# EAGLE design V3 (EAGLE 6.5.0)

## Sheet 1 of 3: FET+Driver
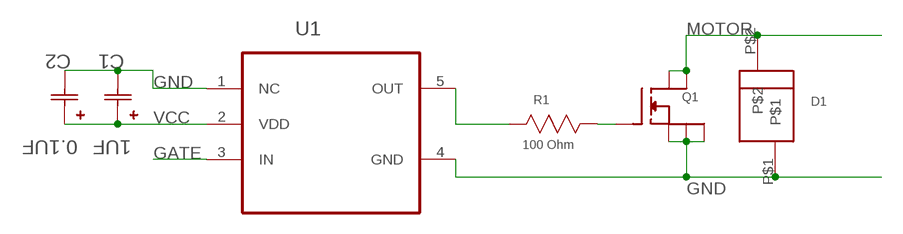
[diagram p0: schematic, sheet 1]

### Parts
C1  1UF  1206YC105KAT2A  [CAPC3216X127N]
C2  0.1UF  0603YC104K4T4A  [CAPC1608X90N]
D1  5.0SMDJ24ASMD  [DO-214AB]
Q1  PSMN039LFPAC  [LFPAC]
R1  100 Ohm  ERA-3AEB101V  [RESC1608X60N]
U1  NCS2001SN1T1G  [SOT95P275X110-5N]

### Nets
GATE: U1.3(IN) ; also sheet 3
GND: C1.2(C2) C2.2(C2) D1.P$1 Q1.1(S1) Q1.2(S2) Q1.3(S3) U1.1(NC) U1.4(GND) ; also sheet 2,3
MOTOR: D1.P$2 Q1.5(D1) Q1.6(D2) ; also sheet 3
N$1: Q1.4(G) R1.1(R1)
N$2: R1.2(R2) U1.5(OUT)
VCC: C1.1(C1) C2.1(C1) U1.2(VDD) ; also sheet 2

## Sheet 2 of 3: Control Power
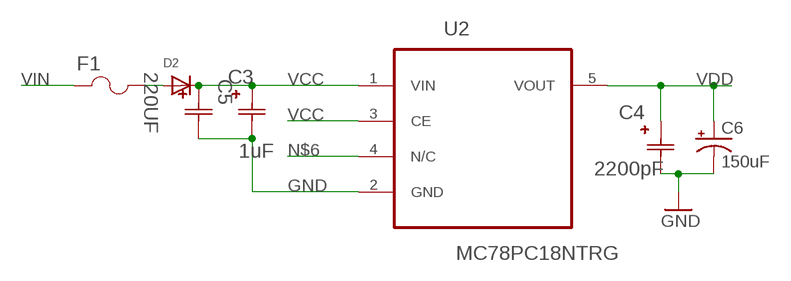
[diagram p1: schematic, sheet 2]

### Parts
C3  1uF  0603YC105KAT2A  [CAPC1608X94N]
C4  2200pF  06033C222JAT4A  [CAPC1608X90N]
C5  220UF  TAJD227K006RNJ  [CAPCP7343X430N]
C6  150uF  47UF-10V-10%(TANT)  [EIA3528]
D2  DIODESOD-123  [SOD-123]
F1  F1206B3R00FWTR  [FUSM3216X140N]
U2  MC78PC18NTRG  [SOT95P275X110-5N]

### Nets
GND: C3.2(C2) C4.2(C2) C5.2(C2) C6.C(-) U2.2(GND) ; also sheet 1,3
N$3: D2.A F1.2
N$6: U2.4(N/C)
VCC: C3.1(C1) C5.1(C1) D2.C U2.1(VIN) U2.3(CE) ; also sheet 1
VDD: C4.1(C1) C6.A(+) U2.5(VOUT) ; also sheet 3
VIN: F1.1

## Sheet 3 of 3: Control + Sensors
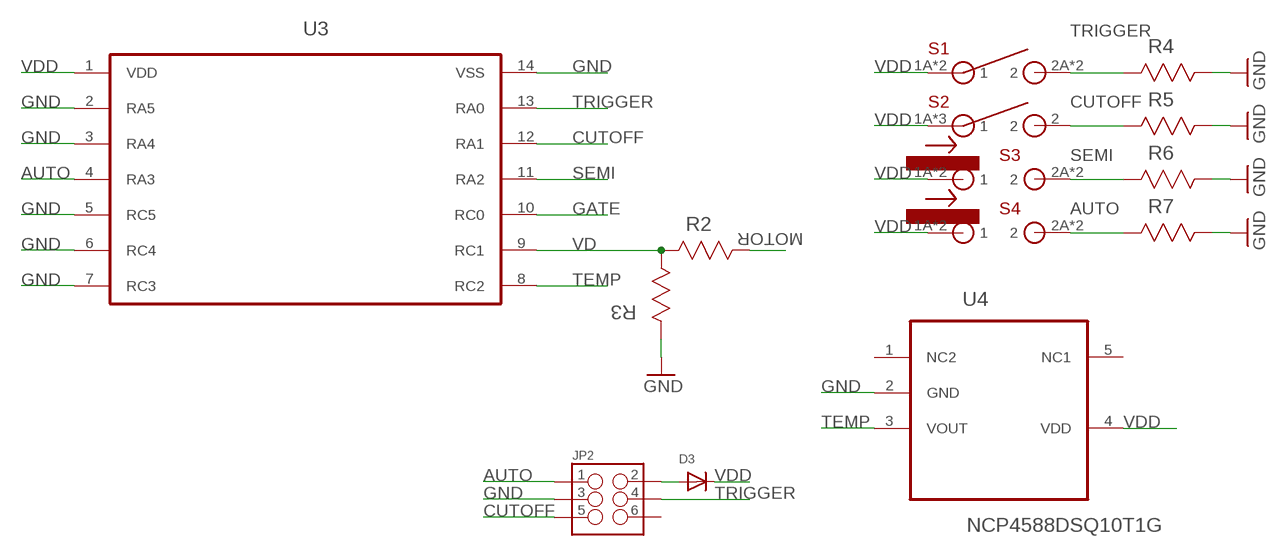
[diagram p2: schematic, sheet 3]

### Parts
D3  DIODESOD-123  [SOD-123]
JP2  M03X2  [2X3_SMD]
R2  15 kOhm  ERA-3AEB153V  [RESC1608X60N]
R3  4.7 kOhm  ERA-3AEB472V  [RESC1608X60N]
R4  4.7 kOhm  ERA-3AEB472V  [RESC1608X60N]
R5  4.7 kOhm  ERA-3AEB472V  [RESC1608X60N]
R6  4.7 kOhm  ERA-3AEB472V  [RESC1608X60N]
R7  4.7 kOhm  ERA-3AEB472V  [RESC1608X60N]
S1  7914S-1-000E  [7914S-1-000E]
S2  ESE-31L15T  [ESE-31L15T]
S3  SPVM110100  [SPVM110100]
S4  SPVM110100  [SPVM110100]
U3  P89LPC912FDH,129  [SOP65P640X110-14N]
U4  NCP4588DSQ10T1G  [SOT65P210X110-5N]

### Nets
AUTO: JP2.1 R7.2(R2) S4.2A S4.2B U3.4(RA3)
CUTOFF: JP2.5 R5.2(R2) S2.2 U3.12(RA1)
GATE: U3.10(RC0) ; also sheet 1
GND: JP2.3 R3.2(R2) R4.1(R1) R5.1(R1) R6.1(R1) R7.1(R1) U3.2(RA5) U3.3(RA4) U3.5(RC5) U3.6(RC4) U3.7(RC3) U3.14(VSS) U4.2(GND) ; also sheet 1,2
MOTOR: R2.1(R1) ; also sheet 1
N$7: D3.A JP2.2
SEMI: R6.2(R2) S3.2A S3.2B U3.11(RA2)
TEMP: U3.8(RC2) U4.3(VOUT)
TRIGGER: JP2.4 R4.2(R2) S1.2A S1.2B U3.13(RA0)
VD: R2.2(R2) R3.1(R1) U3.9(RC1)
VDD: D3.C S1.1A S1.1B S2.1A S2.1B S2.1C S3.1A S3.1B S4.1A S4.1B U3.1(VDD) U4.4(VDD) ; also sheet 2
Unconnected: JP2.6 U4.5(NC1)

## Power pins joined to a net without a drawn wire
NC2: U4.1(NC2)

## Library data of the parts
C1 = AVX_By_element14_Batch_1:1206YC105KAT2A: Capacitor 1206; MPN: 1206YC105KAT2A; OC_FARNELL: 499717; OC_NEWARK: 25C3294; SUPPLIER: AVX; TOLERANCE: ±10%; VOLTAGERATING: 16V
C2 = AVX_By_element14_Batch_1:0603YC104K4T4A: Capacitor, 0603; MPN: 0603YC104K4T4A; OC_FARNELL: 1833863; OC_NEWARK: 85R5663; SUPPLIER: AVX; TOLERANCE: ±10%; VOLTAGERATING: 16V
C3 = AVX_By_element14_Batch_1:0603YC105KAT2A: Capacitor 0603; MPN: 0603YC105KAT2A; OC_FARNELL: 1658870; OC_NEWARK: 96M1178; SUPPLIER: AVX; TOLERANCE: ±10%; VOLTAGERATING: 16V
C4 = AVX_By_element14_Batch_1:06033C222JAT4A: CAPACITOR , 0603; MPN: 06033C222JAT4A; OC_FARNELL: -; OC_NEWARK: 55J3954; SUPPLIER: AVX; TOLERANCE: ±5%; VOLTAGERATING: 25V
C5 = AVX_By_element14_Batch_1:TAJD227K006RNJ: Tantalum Capacitor , 2917; CAPACITANCETOLERANCE: ±10%; MPN: TAJD227K006RNJ; OC_FARNELL: 1658172; OC_NEWARK: 15P3076; SUPPLIER: AVX; VOLTAGERATING: 6.3V
C6 = SparkFun-Capacitors:47UF-10V-10%(TANT): CAP-08310; PROD_ID: CAP-08310; VALUE: 47uF
D1 = custom1:5.0SMDJ24A
D2 D3 = adafruit:DIODE: Diode
F1 = AVX_By_element14_Batch_1:F1206B3R00FWTR: FUSE 2.00A 63V FAST THIN 1206; MPN: F1206B3R00FWTR; OC_FARNELL: 1514506; OC_NEWARK: 05H4220; PACKAGE: 1206; SUPPLIER: AVX
JP2 = SparkFun-Connectors:M03X2: 2x3 .1" header. Shrouded, with keying- CONN-10681 SMT- CONN-11415 Pogo pins- HW-11044; PROD_ID: CONN-11290
Q1 = lfpak mosfet:PSMN039: N-channel LFPAK 100 V 39.5 mΩ standard level MOSFET PSMN039-100YS General description Standard level N-channel MOSFET in LFPAK package qualified to 175 °C. This product is designed and qualified for use in a wide range of industrial, communications and domestic equipment. Features and benefits -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; MPN: PSMN0R9-25YLC,115; OC_FARNELL: 1845636; PACKAGE: LFPAC; SUPPLIER: NXP
R1 = Panasonic_By_element14_Batch_1:ERA-3AEB101V: RESISTOR, 0603; MPN: ERA-3AEB101V; OC_FARNELL: 1577593; OC_NEWARK: 08N2093; SUPPLIER: Panasonic; TOLERANCE: ±0.1%; WATTAGE: 0.1 W
R2 = Panasonic_By_element14_Batch_1:ERA-3AEB153V: RESISTOR, 0603; MPN: ERA-3AEB153V; OC_FARNELL: 1811358; OC_NEWARK: 08N2103; SUPPLIER: Panasonic; TOLERANCE: ±0.1%; WATTAGE: 0.1 W
R3-R7 = Panasonic_By_element14_Batch_1:ERA-3AEB472V: RESISTOR, 0603; MPN: ERA-3AEB472V; OC_FARNELL: 1811387; OC_NEWARK: 08N2126; SUPPLIER: Panasonic; TOLERANCE: ±0.1%; WATTAGE: 0.1 W
S1 = custom1:7914S-1-000E
S2 = custom1:ESE-31L15T
S3 S4 = custom1:SPVM110100
U1 = Banshee:NCS2001SN1T1G: Operational Amplifier; MPN: NCS2001SN1T1G; OC_FARNELL: 1364638; OC_NEWARK: 45J1978; PACKAGE: SOT-23-5; SUPPLIER: ON SEMICONDUCTOR
U2 = ON Semiconductor_By_element14_Batch_1:MC78PC18NTRG: Linear Voltage Regulator; MPN: MC78PC18NTRG; OC_FARNELL: 1130695; OC_NEWARK: 88H4756; PACKAGE: SOT-23-5; SUPPLIER: ON SEMICONDUCTOR
U3 = Banshee:P89LPC912FDH,129: 8-bit microcontrollers with two-clock 80C51 core, 1 kB 3 V flash with 128-byte RAM; MPN: P89LPC912FDH,129; OC_FARNELL: -; OC_NEWARK: 70R8555; PACKAGE: TSSOP-14; SUPPLIER: NXP
U4 = Banshee:NCP4588DSQ10T1G: Linear Voltage Regulator; MPN: NCP4588DSQ10T1G; OC_FARNELL: 1885130; OC_NEWARK: 41T0735; PACKAGE: SC70-5; SUPPLIER: ON SEMICONDUCTOR

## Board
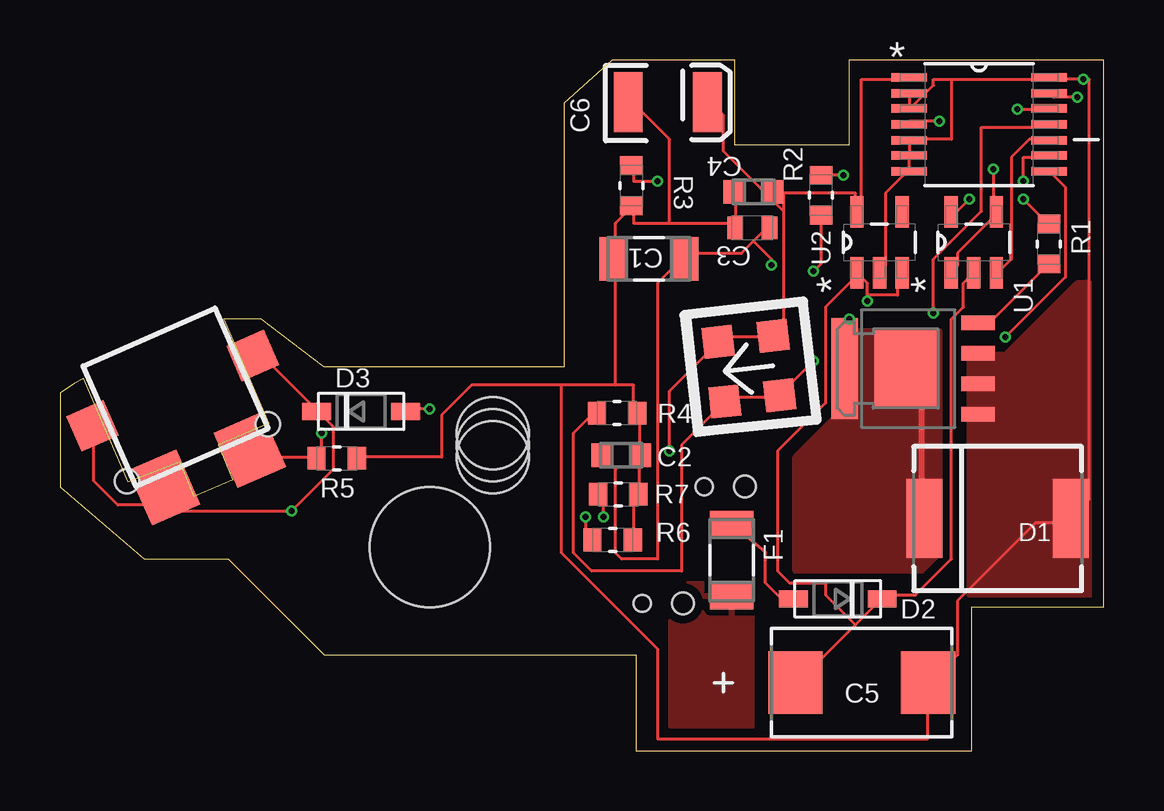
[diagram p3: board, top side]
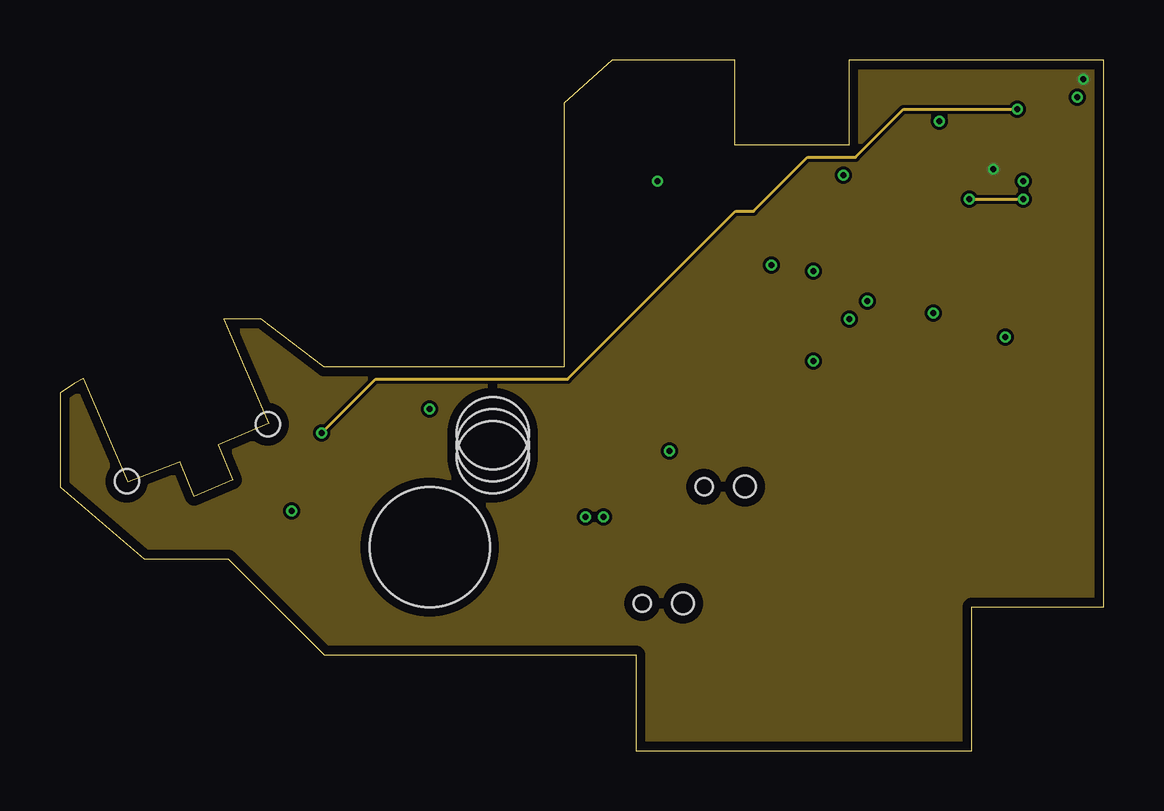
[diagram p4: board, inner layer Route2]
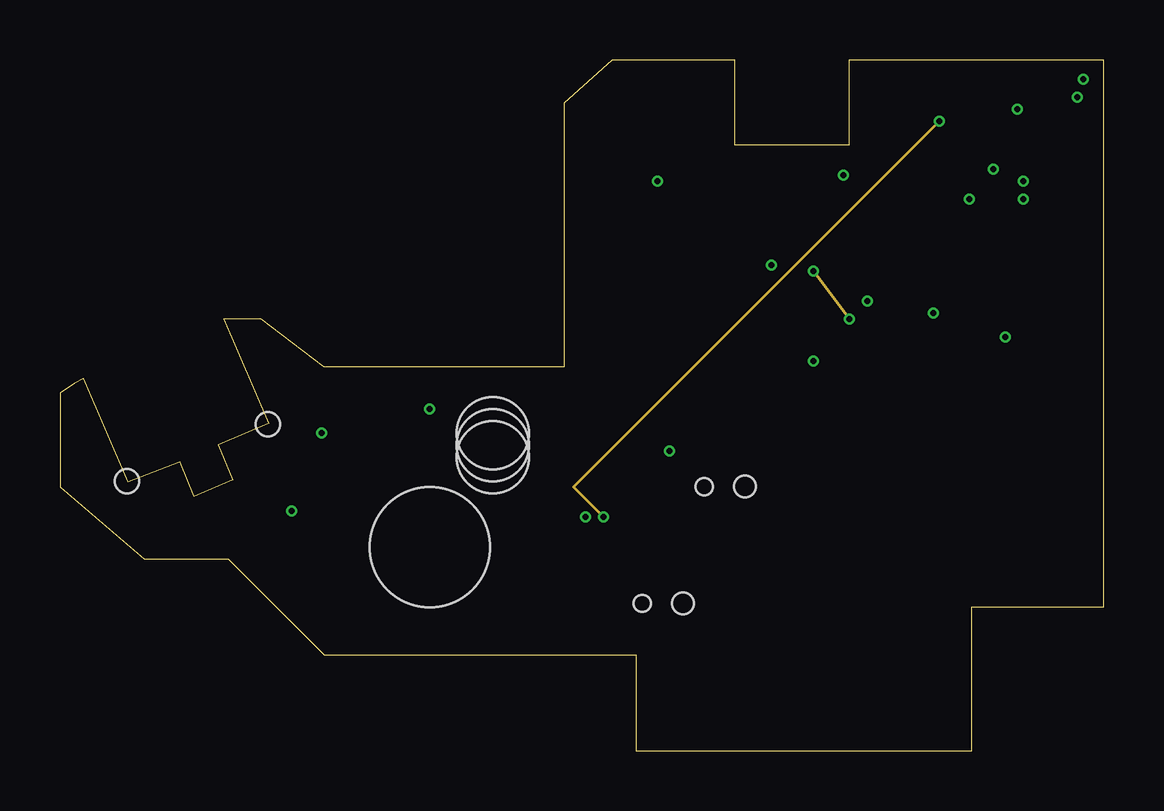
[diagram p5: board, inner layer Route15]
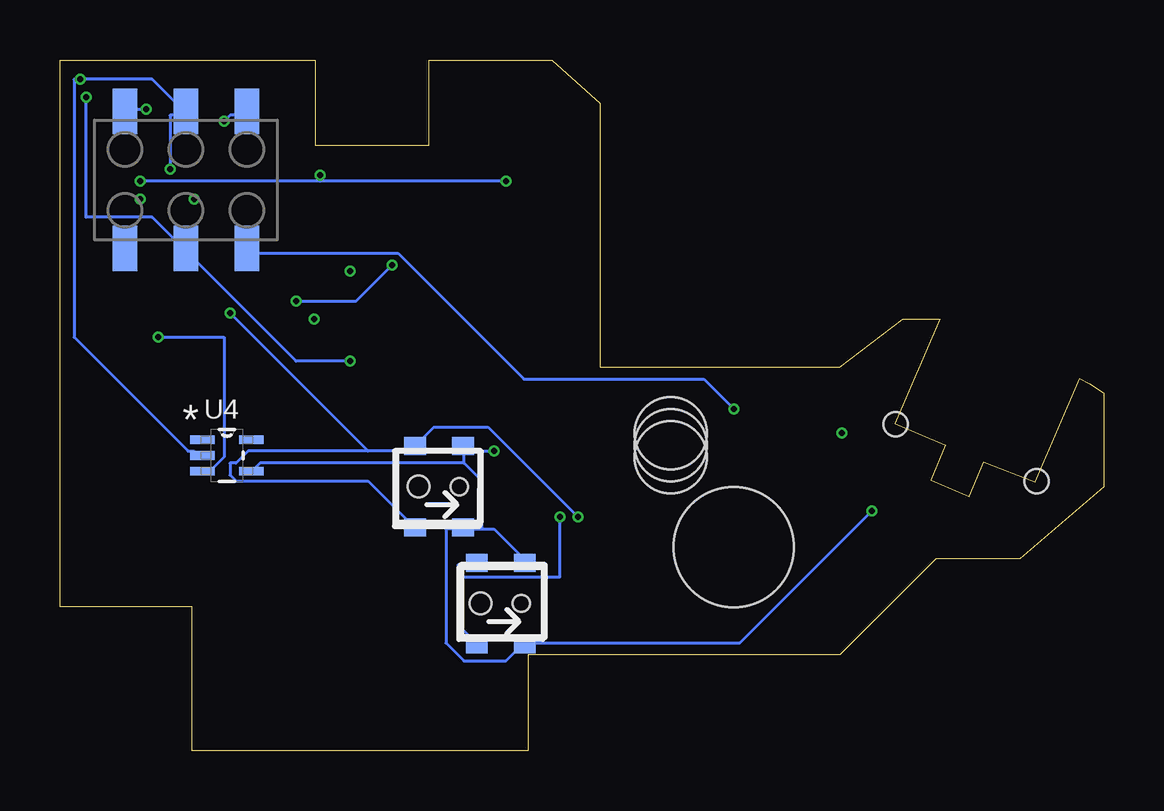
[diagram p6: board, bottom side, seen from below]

Size 43.5 x 28.8 mm. Coordinates in mm from the lower left corner, seen from the top.
Outline: 0,11 3.5,8 7,8 11,4 24,4 24,0 38,0 38,6 43.5,6 43.5,28.8 32.88,28.8 32.88,25.25 28.12,25.25 28.12,28.8 23,28.8 21,27 21,16 11,16 8.38,18 6.82,18 8.7,13.65 6.6,12.75 7.2,11.3 5.6,10.6 5,12.05 2.85,11.2 0.98,15.53 0.6,15.3 0,14.93 0,11
Copper layers (1*2*15*16): Top 0.035559375mm / dielectric 0.17018125mm / Route2 0.01778125mm / dielectric 47mil / Route15 0.01778125mm / dielectric 0.17018125mm / Bottom 0.035559375mm
Design rules "OSHPark-4layer *": minimum track width 5mil, minimum drill 10mil, track to track 5mil, track to pad 5mil, pad to pad 5mil, via to via 5mil, smd to smd 5mil, copper to edge 15mil, drill to drill 6mil, minimum pad ring 4mil, minimum via ring 4mil, stop-mask expansion 4mil, vias tented up to drill 26mil, thermal gap 10mil
Holes 5 mm at 15.41,8.49
Holes 3 mm at 18.04,12.74 18.04,12.24 18.04,13.24
Holes 1 mm at 2.79,11.24 8.66,13.62
bKeepout: area 24,0 to 38,1.5; area 38.5,6 to 43.5,28.8; area 20.4,13.5 to 43.4,29; area -0.1,1.5 to 22.9,19

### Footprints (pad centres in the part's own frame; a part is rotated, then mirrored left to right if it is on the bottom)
CAPC3216X127N = smd 1.118 x 1.803: 1 -1.499,0; 2 1.499,0
CAPC1608X90N = smd 0.864 x 0.965: 1 -0.813,0; 2 0.813,0
CAPC1608X94N = smd 0.66 x 0.94: 1 -0.711,0; 2 0.711,0
CAPCP7343X430N = smd 2.261 x 2.591: 1 -2.769,0; 2 2.769,0
EIA3528 = smd 1.2 x 2.5: A 1.65,0; C -1.65,0
DO-214AB = smd 1.5 x 3.3: P$1 -3.05,0; P$2 3.05,0
SOD-123 = smd 1.2 x 0.7: A 1.85,0; C -1.85,0
FUSM3216X140N = smd 1.118 x 1.803: 1 -1.499,0; 2 1.499,0
2X3_SMD = smd 1.02 x 1.9: 1 -2.54,-2.85; 2 -2.54,2.85; 3 0,-2.85; 4 0,2.85; 5 2.54,-2.85; 6 2.54,2.85
LFPAC = smd 0.6 x 1.4: 1 -1.905,-2.945; 2 -0.635,-2.945; 3 0.635,-2.945; 4 1.905,-2.945 | smd 4.2 x 1.1: 5 0,2.625 | smd 3.3 x 2.7: 6 0,0.025
RESC1608X60N = smd 0.762 x 0.94: 1 -0.838,0; 2 0.838,0
7914S-1-000E = smd 1.3 x 1.25: 1A -1.252,1.151; 1B -1.252,-1.151; 2A 1.252,1.151; 2B 1.252,-1.151
ESE-31L15T = smd 1.7 x 1.6: 1A -3.65,1.3; 1B 3.65,1.3 | smd 2.2 x 2.5: 1C -1.95,-2.25; 2 1.95,-2.25
SPVM110100 = smd 0.75 x 0.9: 1A -1.7,1; 1B 1.7,1; 2A -1.7,-1; 2B 1.7,-1 | hole 0.9: 0,-0.85 | hole 0.7: 0,0.85
SOT95P275X110-5N = smd 1.321 x 0.559: 1 -1.27,0.94; 2 -1.27,0; 3 -1.27,-0.94; 4 1.27,-0.94; 5 1.27,0.94
SOP65P640X110-14N = smd 1.473 x 0.356: 1 -2.921,1.956; 2 -2.921,1.295; 3 -2.921,0.66; 4 -2.921,0; 5 -2.921,-0.66; 6 -2.921,-1.295; 7 -2.921,-1.956; 8 2.921,-1.956; 9 2.921,-1.295; 10 2.921,-0.66; 11 2.921,0; 12 2.921,0.66; 13 2.921,1.295; 14 2.921,1.956
SOT65P210X110-5N = smd 1.016 x 0.356: 1 -1.016,0.66; 2 -1.016,0; 3 -1.016,-0.66; 4 1.016,-0.66; 5 1.016,0.66

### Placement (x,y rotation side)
C1  24.55,20.51 180 top
C2  23.4,12.32 0 top
C3  28.86,21.8 180 top
C4  28.91,23.3 180 top
C5  33.42,2.84 0 top
C6  25.34,27.03 0 top
D1  39.09,9.68 180 top
D2  32.42,6.33 180 top
D3  12.55,14.15 0 top
F1  28,7.95 90 top
JP2  38.25,23.8 180 bottom
Q1  35.33,15.93 90 top
R1  41.22,21.13 90 top
R2  31.72,23.16 90 top
R3  23.82,23.56 270 top
R4  23.22,14.08 180 top
R5  11.54,12.19 180 top
R6  23.04,8.79 180 top
R7  23.27,10.69 180 top
S1  28.72,15.93 276.4 top
S2  5.22,13.82 23.7 top
S3  27.7,11.01 270 bottom
S4  25.12,6.14 270 bottom
U1  38.09,21.2 90 top
U2  34.16,21.2 90 top
U3  38.31,26.11 0 top
U4  36.54,12.31 0 bottom

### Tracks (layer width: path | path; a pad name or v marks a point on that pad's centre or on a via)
AUTO  (via drill 0.25)
  Top 0.127: v36.66,26.24 35.41,26.24 U3.4 | v22.66,9.74 22.66,10.49 R7.2
  Route15 0.127: v36.66,26.24 21.41,10.99 v22.66,9.74
  Bottom 0.127: v36.66,26.24 36.41,26.49 35.91,26.49 JP2.1 | 26.91,7.24 26.91,7.74 26.16,7.74 S4.2A | 26.91,7.24 26.91,5.24 26.16,4.49 S4.2B | v22.66,9.74 22.66,7.24 26.91,7.24
CUTOFF  (via drill 0.25)
  Top 0.127: v39.91,26.74 41.16,26.74 U3.12 | S2.2 7.91,12.49 7.91,12.24 10.66,12.24 R5.2 10.91,12.24 v10.91,13.24
  Route2 0.127: v39.91,26.74 35.16,26.74 33.16,24.74 31.16,24.74 28.91,22.49 28.16,22.49 21.16,15.49 13.16,15.49 v10.91,13.24
  Bottom 0.127: v39.91,26.74 40.66,26.74 JP2.5
GATE
  Top 0.127: U1.3 39.16,19.99 39.66,20.49 39.66,24.74 40.41,25.49 41.16,25.49 U3.10
GND  (via drill 0.25)
  Top 0.127: C4.2 28.16,23.24 28.16,21.99 C3.2 27.91,21.99 25.41,21.99 | 25.41,21.99 23.91,21.99 23.91,22.49 R3.2 23.66,22.49 23.16,21.99 23.16,20.74 C1.2 23.16,20.49 23.16,15.24 | 25.41,21.99 25.41,25.49 23.91,26.99 C6.C | R6.1 23.91,8.99 23.91,10.49 R7.1 24.16,10.74 24.16,12.24 C2.2 24.16,12.49 24.16,13.99 R4.1 23.91,14.24 23.91,15.24 23.16,15.24 | 23.16,15.24 20.91,15.24 | 20.91,15.24 17.16,15.24 15.91,13.99 15.91,12.24 12.41,12.24 R5.1 | U1.1 37.16,19.99 37.41,20.24 37.41,20.74 38.91,22.24 U1.4 38.91,22.49 v38.91,24.24 | 35.41,25.49 35.41,24.99 U3.6 35.41,24.74 35.41,24.24 U3.7 35.16,23.99 34.41,23.24 34.41,20.24 34.16,19.99 U2.2 | 35.41,26.74 35.41,27.24 U3.2 | 37.16,27.99 36.41,27.99 36.41,27.74 35.41,26.74 | 37.16,27.99 41.16,27.99 U3.14 41.41,27.99 v42.66,27.99 42.91,27.99 42.91,10.49 42.16,9.74 D1.P$1 41.91,9.49 40.66,9.49 37.41,6.24 37.41,3.99 36.41,2.99 C5.2 36.16,2.74 36.16,0.49 24.91,0.49 24.91,4.24 20.91,8.24 20.91,15.24 | 35.41,26.74 U3.3 | 35.41,25.49 37.16,25.49 37.16,27.99 | 35.41,25.49 U3.5
  Bottom 0.127: U4.2 37.66,12.24 37.91,12.49 38.16,12.49 42.91,17.24 42.91,27.99 v42.66,27.99 39.66,27.99 38.41,26.74 JP2.3 38.41,26.49 38.91,26.49 v38.91,24.24
  pour Route2: -1.09,29.49 43.91,29.49 43.91,-1.01 -1.09,-1.01
  pour Top (no thermals): 39.41,16.49 37.91,16.49 37.91,6.49 42.91,6.49 42.91,19.49 42.41,19.49
MOTOR  (via drill 0.25)
  Top 0.127: R2.1 31.72,20.3 v31.41,19.99 | Q1.5 32.7,17.79 v32.91,17.99
  Top 0.254: Q1.6 35.91,15.93 35.91,9.49
  Route15 0.127: v32.91,17.99 v31.41,19.99
  pour Top (no thermals): 32.41,17.49 36.66,17.49 36.66,8.24 35.91,7.49 30.66,7.49 30.66,12.24 32.41,13.99
N$1
  Top 0.127: R1.1 41.16,20.24 38.91,17.99 38.41,17.99 Q1.4
N$2  (via drill 0.25)
  Top 0.127: v40.16,22.99 41.16,21.99 R1.2 | v37.91,22.99 37.16,22.24 U1.5
  Route2 0.127: v37.91,22.99 v40.16,22.99
N$3
  Top 0.127: D2.A 30.41,6.24 30.16,6.24 29.41,6.99 29.41,8.29 F1.2
N$7  (via drill 0.25)
  Top 0.127: v15.41,14.24 14.41,14.24 D3.A
  Bottom 0.127: v15.41,14.24 16.66,15.49 24.16,15.49 29.41,20.74 35.66,20.74 JP2.2
SEMI  (via drill 0.25)
  Top 0.127: v21.91,9.74 21.91,9.24 22.16,8.99 R6.2 | v36.41,18.24 36.41,20.49 38.41,22.49 38.41,25.99 41.16,25.99 U3.11
  Bottom 0.127: 30.66,12.49 28.91,12.49 S3.2A 28.66,12.74 27.91,13.49 25.66,13.49 v21.91,9.74 | 30.66,12.49 35.66,12.49 36.16,11.99 36.41,11.99 36.41,11.49 36.16,11.24 30.66,11.24 28.91,9.49 S3.2B | 30.66,12.49 v36.41,18.24
TEMP  (via drill 0.25)
  Top 0.127: v39.41,17.24 41.91,19.74 41.91,23.49 41.41,23.99 U3.8
  Bottom 0.127: v39.41,17.24 36.66,17.24 36.66,12.24 37.16,11.74 37.41,11.74 U4.3
TRIGGER  (via drill 0.25)
  Top 0.127: v42.41,27.24 41.41,27.24 U3.13 | R4.2 22.16,13.99 21.41,13.24 21.41,8.24 22.16,7.49 25.91,7.49 25.91,12.74 27.66,14.49 S1.2B 27.91,14.74 29.91,14.74 S1.2A 30.16,14.99 v31.41,16.24
  Bottom 0.127: v42.41,27.24 42.41,22.24 39.66,22.24 38.41,20.99 JP2.4 38.16,20.74 33.66,16.24 v31.41,16.24
VCC  (via drill 0.25)
  Top 0.127: 28.91,21.24 28.41,20.74 26.16,20.74 C1.1 25.91,20.49 24.91,19.49 24.91,7.99 23.41,7.99 23.16,8.24 23.16,11.74 22.66,12.24 C2.1 | 28.91,21.24 29.41,21.74 C3.1 | 33.66,18.99 33.66,19.49 33.41,19.74 U2.1 33.16,19.74 31.91,18.49 31.91,14.49 29.91,12.49 29.91,7.49 30.41,6.99 31.91,6.99 31.91,6.49 33.16,5.24 | 33.66,18.99 34.91,18.99 34.91,19.74 U2.3 | 33.16,5.24 30.66,2.74 C5.1 | 33.16,5.24 34.16,6.24 D2.C 34.41,6.49 35.66,6.49 37.16,7.99 37.16,17.99 37.66,18.49 37.66,19.49 37.91,19.74 U1.2 | 28.91,21.24 29.66,20.49 v29.66,20.24 | 33.66,18.99 v33.66,18.74
  Bottom 0.127: v29.66,20.24 31.16,18.74 v33.66,18.74
VD  (via drill 0.25)
  Top 0.127: 23.66,24.49 R3.1 23.91,24.24 23.91,23.74 v24.91,23.74 | v40.16,23.74 40.16,24.74 41.16,24.74 U3.9 | v32.66,23.99 31.91,23.99 R2.2
  Bottom 0.127: v24.91,23.74 32.66,23.74 | 32.66,23.74 v40.16,23.74 | 32.66,23.74 v32.66,23.99
VDD  (via drill 0.25)
  Top 0.127: 30.16,23.24 33.16,23.24 33.16,22.49 U2.5 33.41,22.49 33.41,27.99 35.16,27.99 U3.1 | 30.16,23.24 29.91,23.24 C4.1 | 30.16,23.24 30.16,22.49 | 30.16,22.49 30.16,17.74 29.91,17.49 S1.1A 29.66,17.24 27.66,17.24 S1.1B 27.41,16.99 25.41,14.99 v25.41,12.49 | 30.16,22.49 27.66,24.99 27.66,26.49 27.16,26.99 C6.A | S2.1B 8.16,16.24 8.66,16.24 10.66,14.24 D3.C 10.91,13.99 11.41,13.49 11.41,11.74 v9.66,9.99 4.16,9.99 4.16,10.24 | 4.16,10.24 2.41,10.24 1.41,11.24 1.41,13.24 1.16,13.49 S2.1A | 4.16,10.24 4.16,10.74 S2.1C 4.16,10.24
  Bottom 0.127: 25.91,9.24 26.66,9.24 S3.1B 26.91,9.24 27.41,9.24 27.41,4.49 26.66,3.74 24.91,3.74 24.16,4.49 S4.1B 23.91,4.49 15.16,4.49 v9.66,9.99 | 25.91,9.24 25.41,9.24 24.16,7.99 S4.1A | 26.66,11.99 26.66,12.49 | 26.66,11.99 25.91,11.24 25.91,9.24 | 26.66,11.99 35.16,11.99 35.41,11.74 U4.4 | 26.66,12.49 v25.41,12.49 | 26.66,12.49 S3.1A
VIN
  pour Top: 28.91,0.99 28.91,6.99 25.41,6.99 25.41,0.99

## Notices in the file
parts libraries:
SparkFun-Capacitors: Licensing: Creative Commons ShareAlike 4.0 International - https://creativecommons.org/licenses/by-sa/4.0
